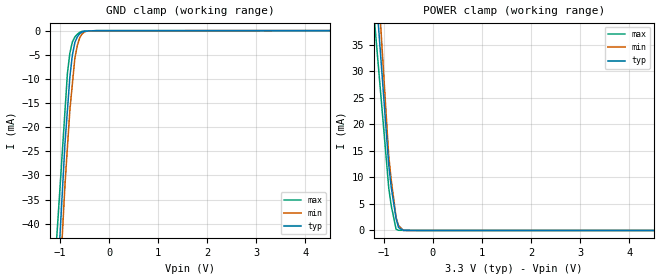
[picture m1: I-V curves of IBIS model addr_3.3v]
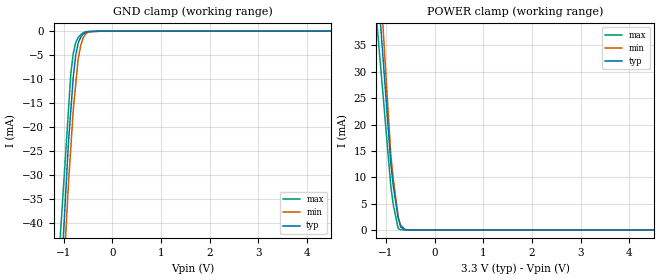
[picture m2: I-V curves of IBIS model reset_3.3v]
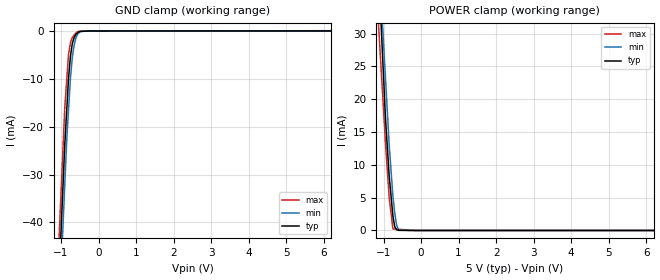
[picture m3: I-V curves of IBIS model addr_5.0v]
| Teraspeed Modeling Services.
| http://www.teraspeed.com
[IBIS Ver]   4.2
[Comment Char] |_char
[File Name]   pca9646pw.ibs
[File Rev]   3.0
[Source]  Measured and created by Teraspeed Consulting Group LLC
[Date]   02-07-2013
[Notes]   Quality Check of this IBIS model: Model Passes IBIS Check
   Model parses into ICX IS. Simulation done with Hyperlynx.
   1. MIN TYP MAX information is based on Temperature and Voltage
   characteristics only.
   2. Package data gained using Tektronix IConnect Software.
[Disclaimer]
| Use: Teraspeed Consulting Group LLC ("Teraspeed") has
| licensed IBIS models to specific integrated circuit
| suppliers ("IC Vendors") for use and distribution as
| follows: Each IC Vendor may use IBIS Models, and distribute
| them to IC Vendor's customers to use solely for developing
| printed circuit board designs. Users of this model may
| modify the IBIS model to suit its specific applications but
| rights to derivative works and such modifications shall belong
| to Teraspeed. No other distribution of these materials is
| permitted.
| DISCLAIMER OF WARRANTY: UNLESS OTHERWISE AGREED TO IN WRITING
| TERASPEED DISCLAIMS AND USER WAIVES ALL WARRANTIES, EXPRESS
| OR IMPLIED, INCLUDING WARRANTIES OF MERCHANTABILITY AND
| FITNESS FOR A PARTICULAR PURPOSE. IN NO EVENT SHALL
| TERASPEED BE LIABLE FOR ANY DIRECT OR INDIRECT DAMAGES,
| WHETHER IN CONTRACT OR TORT, INCLUDING, WITHOUT LIMITATION,
| LOST PROFITS, BUSINESS INTERRUPTION, OR LOST INFORMATION
| ARISING OUT OF THE USE OF OR THE INABILITY TO USE THE MODEL,
| EVEN IF TERASPEED HAS BEEN ADVISED OF THE POSSIBILITY OF SUCH
| DAMAGES.
[Copyright]
| This file is the legal property of Teraspeed Copyright(c) 2013.
| All other rights are reserved.
[Component] PCA9646PW
[Manufacturer] NXP Semiconductors
[Package]
| TSSOP16/SOT403-1
| variable  typ   min   max
R_pkg   1.000E-02  1.000E-02  1.000E-02
L_pkg   1.918E-09  1.790E-09  2.090E-09
C_pkg   5.640E-13  4.800E-13  6.840E-13
[Pin] signal_name  model_name  R_pin  L_pin C_pin
1   A0   addr_in   1.000E-02 2.090E-09 6.840E-13
2   A1   addr_in   1.000E-02 1.960E-09 5.920E-13
3   *RESET  reset_in  1.000E-02 1.830E-09 5.000E-13
4   SD0   io_od   1.000E-02 1.790E-09 4.800E-13
5   SC0   io_od   1.000E-02 1.790E-09 4.800E-13
6   SD1   io_od   1.000E-02 1.830E-09 5.000E-13
7   SC1   io_od   1.000E-02 1.960E-09 5.920E-13
8   VSS   GND   1.000E-02 2.090E-09 6.840E-13
9   SD2   io_od   1.000E-02 2.090E-09 6.840E-13
10   SC2   io_od   1.000E-02 1.960E-09 5.920E-13
11   SD3   io_od   1.000E-02 1.830E-09 5.000E-13
12   SC3   io_od   1.000E-02 1.790E-09 4.800E-13
13   A2   addr_in   1.000E-02 1.790E-09 4.800E-13
14   SCL   io_od   1.000E-02 1.830E-09 5.000E-13
15   SDA   io_od   1.000E-02 1.960E-09 5.920E-13
16   VDD   POWER   1.000E-02 2.090E-09 6.840E-13
[Model Selector] addr_in
addr_3.3v   i2c address pin,vdd=3.3v
addr_5.0v   i2c address pin,vdd=5.0v
[Model Selector] reset_in
reset_3.3v  reset pin,vdd=3.3v
reset_5.0v  reset pin,vdd=5.0v
[Model Selector] io_od
io_od_3.3v  open drain io pin,vdd=3.3v
io_od_5.0v  open drain io pin,vdd=5.0v
| Models and submodels in the file (6): addr_3.3v (Input), reset_3.3v (Input), addr_5.0v (Input), reset_5.0v (Input), io_od_3.3v (I/O_open_drain), io_od_5.0v (I/O_open_drain)
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[Model] addr_3.3v
Model_type Input
Vinl = 700.000mV
Vinh = 1.70000V
C_comp 631.000fF 630.000fF 632.000fF
| variable typ   min   max
[Voltage Range] 3.30000V 2.70000V 3.60000V
[POWER Clamp Reference] 3.30000V 2.70000V 3.60000V
[GND Clamp Reference] 0.00000V 0.00000V 0.00000V
[Temperature Range]   25   85   -40
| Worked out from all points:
|   GND clamp passes 1 mA (typ) near -0.63 V on its own axis
|   POWER clamp passes 1 mA (typ) near -0.71 V on its own axis
[GND Clamp]
-3.3V     -472.2mA   -491.7mA   -392.1mA
-900mV    -23.31mA   -31.86mA   -16.6mA
-850mV    -16.42mA   -24.1mA    -8.773mA
-800mV    -9.519mA   -16.34mA   -4.606mA
-750mV    -5.068mA   -11.07mA   -2.377mA
-700mV    -2.495mA   -5.805mA   -1.317mA
-650mV    -1.298mA   -3.123mA   -767.8uA
-600mV    -631.3uA   -1.45mA    -370.3uA
-550mV    -283.2uA   -636.9uA   -135.2uA
-450mV    -84.32uA   -93.63uA   -88.23uA
-225mV    -6.281uA   -24.99uA   -5.877uA
6.6V      7.519uA    8.9uA      6.122uA
[POWER Clamp]
-3.3V     312.9mA    374.3mA    268.6mA
-1.2V     49.91mA    59.04mA    40.62mA
-1.1V     37.38mA    44.03mA    29.76mA
-1.05V    31.12mA    36.52mA    24.33mA
-900mV    12.34mA    14.01mA    8.039mA
-850mV    8.174mA    9.568mA    4.698mA
-750mV    2.237mA    2.459mA    239uA
-700mV    553.6uA    919.5uA    38.44uA
-600mV    20.46uA    0A         30.75uA
6.6V      0A         0A         0A
[Model] reset_3.3v
Model_type Input
Vinl = 650.000mV
Vinh = 2.00000V
C_comp 695.000fF 691.000fF 699.000fF
| variable typ   min   max
[Voltage Range] 3.30000V 2.70000V 3.60000V
[POWER Clamp Reference] 3.30000V 2.70000V 3.60000V
[GND Clamp Reference] 0.00000V 0.00000V 0.00000V
[Temperature Range]   25   85   -40
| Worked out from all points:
|   GND clamp passes 1 mA (typ) near -0.63 V on its own axis
|   POWER clamp passes 1 mA (typ) near -0.71 V on its own axis
[GND Clamp]
-3.3V     -472.2mA   -491.7mA   -392.1mA
-900mV    -23.31mA   -31.86mA   -16.6mA
-850mV    -16.42mA   -24.1mA    -8.773mA
-800mV    -9.519mA   -16.34mA   -4.606mA
-750mV    -5.068mA   -11.07mA   -2.377mA
-700mV    -2.495mA   -5.805mA   -1.317mA
-650mV    -1.298mA   -3.123mA   -767.8uA
-600mV    -631.3uA   -1.45mA    -370.3uA
-550mV    -283.2uA   -636.9uA   -135.2uA
-450mV    -84.32uA   -93.63uA   -88.23uA
-225mV    -6.281uA   -24.99uA   -5.877uA
6.6V      7.519uA    8.9uA      6.122uA
[POWER Clamp]
-3.3V     312.9mA    374.3mA    268.6mA
-1.2V     49.91mA    59.04mA    40.62mA
-1.1V     37.38mA    44.03mA    29.76mA
-1.05V    31.12mA    36.52mA    24.33mA
-900mV    12.34mA    14.01mA    8.039mA
-850mV    8.174mA    9.568mA    4.698mA
-750mV    2.237mA    2.459mA    239uA
-700mV    553.6uA    919.5uA    38.44uA
-600mV    20.46uA    0A         30.75uA
6.6V      0A         0A         0A
[Model] addr_5.0v
Model_type Input
Vinl = 1.50000V
Vinh = 3.50000V
C_comp 631.000fF 630.000fF 632.000fF
| variable typ   min   max
[Voltage Range] 5.00000V 4.50000V 5.50000V
[POWER Clamp Reference] 5.00000V 4.50000V 5.50000V
[GND Clamp Reference] 0.00000V 0.00000V 0.00000V
[Temperature Range]   25   85   -40
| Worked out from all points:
|   GND clamp passes 1 mA (typ) near -0.62 V on its own axis
|   POWER clamp passes 1 mA (typ) near -0.71 V on its own axis
[GND Clamp]
-5V       -769.3mA   -773.1mA   -750mA
-900mV    -23.68mA   -32.07mA   -15.91mA
-850mV    -16.78mA   -23.03mA   -10.38mA
-800mV    -9.872mA   -16.48mA   -4.856mA
-750mV    -5.327mA   -9.922mA   -2.468mA
-700mV    -2.633mA   -5.546mA   -1.35mA
-650mV    -1.363mA   -2.96mA    -865.5uA
-600mV    -657.7uA   -1.366mA   -380.9uA
-550mV    -296uA     -596.3uA   -141uA
-450mV    -89.66uA   -85.33uA   -29.3uA
-225mV    -7.223uA   -6.377uA   -516.8nA
10V       10.81uA    1.638uA    79.28uA
[POWER Clamp]
-5V       517.3mA    443.6mA    409.6mA
-1.25V    54.33mA    54.56mA    42.78mA
-950mV    17.29mA    23.43mA    13.43mA
-850mV    8.325mA    13.06mA    5.028mA
-750mV    2.183mA    5.224mA    235.9uA
-700mV    538uA      2.573mA    217uA
-650mV    106.2uA    762uA      198.1uA
-600mV    20.1uA     126uA      179.3uA
-100mV    0A         0A         0A
10V       0A         0A         0A
